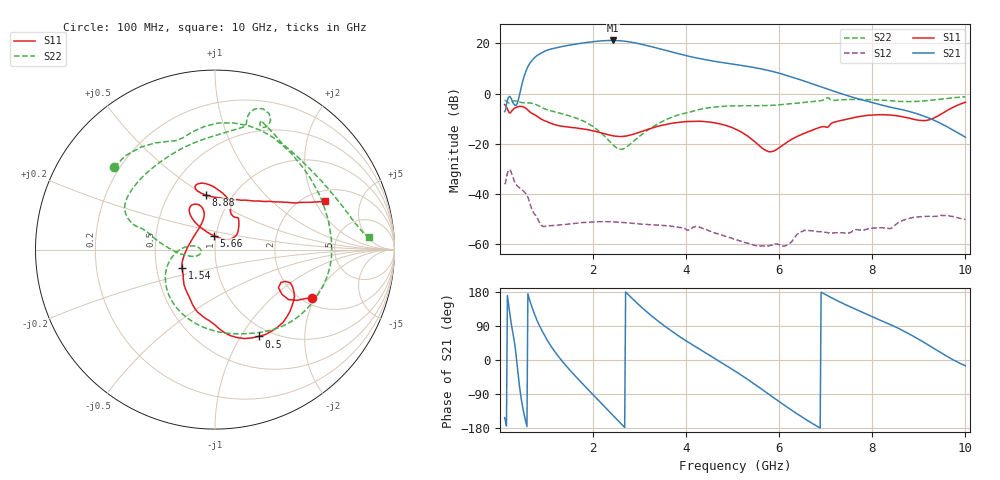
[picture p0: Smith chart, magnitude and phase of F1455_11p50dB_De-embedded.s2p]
! Integrated Device Technology
! Corporate Headquarters
! 6024 Silver Creek Valley Road
! San Jose, CA 95138  USA
! Phone:  1-408-284-8200
! Toll Free:  1-800-223-1366
! Webpage:  http://www.idt.com/
! Timing and RF Division
! 515 Groton Road, Suite 102
! Westford, MA 01886-6024
! Device:  F1455
! Description: 6-bit 0.5 dB Transmit Variable Gain Amplifier
! Frequency:  1400.0 -  2300.00 MHz
! Package:  6x6 mm Thin QFN Plastic Package: 28 pin
! State:  23
! Atten State:  11.5 dB
! Voltage:  +5.00 Volts
! Current:  217.672 mA
! Data:  The device was measured on a the F1455 evaluation board which has
!  individual transmission lines to the RF pins.  Data was collected
!  using a calibrated network analyzer.  The evaluation board was
!  de-embedded using a TRL calibration technique.
!  The reference plane is the edge of the package pin.
!  Pin  1 = CSb
!  Pin  2 = DATA
!  Pin  3 = CLK
!  Pin  4 = RSET
!  Pin  5 = GND
!  Pin  6 = RFIN  = Port 1
!  Pin  7 = GND
!  Pin  8 = NC
!  Pin  9 = NC
!  Pin 10 = NC
!  Pin 11 = NC
!  Pin 12 = NC
!  Pin 13 = NC
!  Pin 14 = /STBY
!  Pin 15 = GND
!  Pin 16 = RFOUT  = Port 2
!  Pin 17 = GND
!  Pin 18 = NC
!  Pin 19 = NC
!  Pin 20 = NC
!  Pin 21 = GND
!  Pin 22 = NC
!  Pin 23 = GND
!  Pin 24 = NC
!  Pin 25 = NC
!  Pin 26 = NC
!  Pin 27 = GND
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# GHz S dB R 50
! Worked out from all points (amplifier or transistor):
!   496 points, 100 MHz to 10 GHz, reference 50 ohm
!   highest |S21| = 21.2 dB at 2.42 GHz (marker M1)
!   |S21| within 3 dB of that: 1.191 GHz to 3.364 GHz (2.172 GHz wide, 95.4 % of centre)
!   unconditionally stable (mu >= 1): start of sweep to end of sweep
!   at 1.74 GHz: K = 16.42, MAG = 20.6 dB, |S12| = -51.6 dB
!   at 5.06 GHz: K = 69.62, MAG = 13.5 dB, |S12| = -58.2 dB
!   at 10 GHz: K = 171.57, MAG = -9.0 dB, |S12| = -50.3 dB
!   S11 on the Smith chart (normalised r, x): 100 MHz: 2.24, -1.89; 500 MHz: 0.87, -1.20; 1.54 GHz: 0.68, -0.15; 5.66 GHz: 0.97, +0.15; 8.88 GHz: 0.76, +0.51; 10 GHz: 2.45, +2.44
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0.1  -4.40 -26.5  -7.24 -152.2  -36.20 45.1  -2.79 140.7
0.38  -5.30 -40.1  -3.49 -25.5  -37.00 -112.9  -3.19 56.9
0.5  -5.33 -63.4  5.68 -132.1  -38.82 -151.2  -3.64 27.9
0.68  -7.83 -92.7  13.03 142.1  -45.95 146.3  -3.85 -14.0
0.8  -9.08 -107.9  15.22 103.6  -49.65 129.5  -4.61 -41.8
0.94  -10.67 -120.9  16.71 69.1  -53.08 124.2  -5.95 -68.0
1.24  -12.73 -140.1  18.40 12.0  -52.55 93.5  -7.63 -109.6
1.54  -13.52 -150.5  19.47 -31.9  -51.98 65.1  -9.17 -140.4
1.76  -14.01 -157.4  20.11 -60.9  -51.54 48.1  -10.72 -158.4
2.1  -15.33 -171.6  20.91 -104.1  -51.18 25.7  -14.57 178.6
2.42  -16.83 164.5  21.20 -145.1  -51.18 7.1  -20.29 171.6
2.6  -17.13 146.3  21.05 -168.0  -51.44 -2.5  -22.25 -173.7
2.78  -16.69 129.2  20.65 169.7  -51.69 -10.8  -20.51 -161.5
3.08  -14.91 111.4  19.52 135.0  -52.23 -22.9  -15.82 -168.2
3.4  -13.05 106.2  18.02 102.4  -52.54 -34.6  -12.04 178.9
4.08  -11.13 114.6  14.78 44.3  -54.24 -53.5  -7.38 163.8
5.06  -14.16 126.1  11.58 -29.9  -58.21 -96.2  -4.90 148.6
5.66  -22.17 95.7  9.66 -80.1  -60.80 -96.1  -4.82 124.4
6.7  -14.70 44.2  3.96 -166.6  -54.81 -138.5  -3.22 78.5
8.36  -8.54 106.7  -5.34 94.7  -53.95 157.1  -2.84 62.5
8.88  -10.25 99.4  -7.62 62.8  -49.47 140.8  -3.19 42.0
10  -3.45 24.0  -17.48 -15.4  -50.25 67.3  -1.29 4.7
